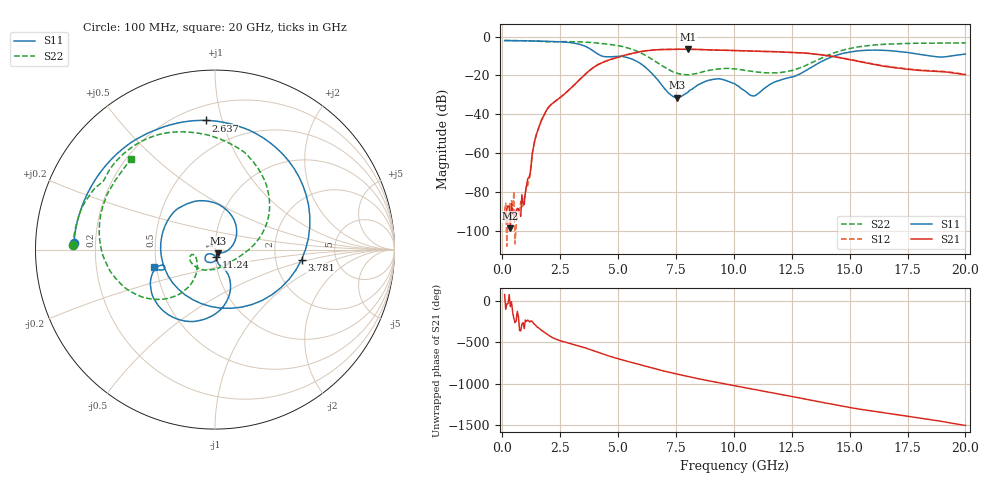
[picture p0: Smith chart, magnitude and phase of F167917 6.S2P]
!  2-Port S-parameters saved by WinCal
! VAR MeasName=S-Parameters (CALIBRATED_DATA) read from VNA (N5242A)
! VAR MeasDate=2016-11-22 8:59:58
! VAR NAME=F167917 6
! VAR FILENAME=F167917 6.S2P
! VAR DATE=2016-11-22 8:59:58
! VAR PHYS_PORTS=1,2
# Hz S DB R 50
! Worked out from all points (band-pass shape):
!   401 points, 100 MHz to 20 GHz, reference 50 ohm
!   highest |S21| = -6.53 dB at 8.01 GHz (marker M1); lowest = -98.7 dB at 348.8 MHz (marker M2)
!   |S21| within 3 dB of the highest: 5.315 GHz to 13.85 GHz (8.536 GHz wide, 89.1 % of centre)
!   lowest |S11| = -31.4 dB at 7.562 GHz (marker M3), VSWR 1.05, Z = 51.8 - j2.03 ohm
!   |S11| at or under -10 dB: 4.289 GHz to 14.34 GHz (10.05 GHz wide, 108 % of centre); 18.48 GHz to 19.4 GHz (919.3 MHz wide, 4.85 % of centre)
!   |S22| runs from -19.8 to -2.0 dB; largest |S21 - S12| = 0.0049
!   S11 on the Smith chart (normalised r, x): 100 MHz: 0.12, +0.02; 2.637 GHz: 0.29, +0.89; 3.781 GHz: 2.82, -0.42; 11.24 GHz: 1.01, -0.09; 20 GHz: 0.48, -0.11
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1e8  -2.09 177.3  -92.97 75.4  -89.98 86.8  -2.03 178.3
3.4875e8  -2.11 170.7  -98.72 -69.8  -84.88 -122.9  -2.06 174.2
9.955e8  -2.22 153.3  -80.20 128.1  -81.16 90.0  -2.17 163.7
1.64225e9  -2.36 134.0  -44.68 17.1  -44.62 16.5  -2.47 153.2
2.63725e9  -2.83 94.2  -30.09 -131.7  -30.12 -131.9  -2.63 138.8
3.43325e9  -4.35 35.9  -21.11 166.8  -21.13 166.8  -2.79 121.9
3.7815e9  -6.27 -6.7  -17.36 135.0  -17.35 135.1  -3.02 113.3
4.1795e9  -9.40 -74.9  -14.23 95.2  -14.17 95.2  -3.46 102.8
4.72675e9  -10.41 -173.6  -11.67 45.3  -11.63 45.0  -4.22 86.9
5.72175e9  -12.26 80.9  -8.38 -32.9  -8.41 -33.1  -7.09 48.3
6.7665e9  -23.14 -4.5  -6.74 -110.5  -6.76 -110.5  -14.02 2.7
7.5625e9  -31.45 -46.8  -6.55 -162.9  -6.57 -162.9  -18.96 -38.3
8.01025e9  -28.73 -62.9  -6.53 169.8  -6.53 169.8  -19.72 -72.0
9.1545e9  -22.00 -116.9  -6.96 104.3  -6.94 104.3  -16.94 -135.6
1.005e10  -24.41 -147.0  -7.21 56.6  -7.22 56.7  -16.73 -162.2
1.079625e10  -30.52 -119.2  -7.52 17.8  -7.50 18.0  -17.98 -167.5
1.1244e10  -27.44 -84.1  -7.64 -5.2  -7.63 -5.0  -18.56 -163.9
1.238825e10  -21.15 -75.0  -8.11 -64.8  -8.10 -64.8  -17.82 -141.0
1.338325e10  -15.61 -62.5  -8.86 -119.0  -8.85 -118.5  -13.31 -125.1
1.51245e10  -7.78 -103.5  -12.19 150.6  -12.08 150.9  -5.87 -150.9
1.67165e10  -7.27 -143.2  -15.64 82.6  -15.57 82.4  -3.87 177.0
2e10  -9.02 -164.2  -19.62 -60.1  -19.49 -60.6  -3.29 132.8
